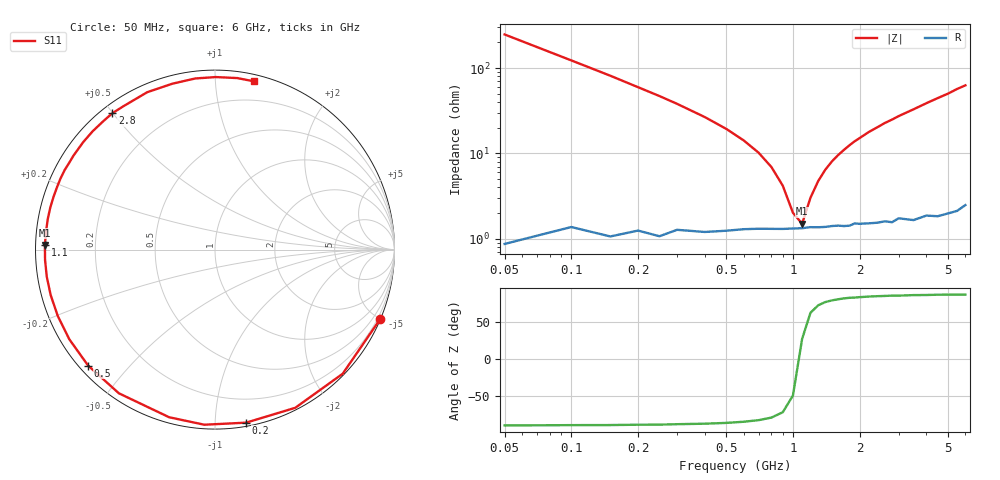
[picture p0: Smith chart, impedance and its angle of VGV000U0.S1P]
! Infineon Technologies  Discrete & RF Semiconductors
! BB 831
! Si Tuning Diode in SOD323
! VR = 0 V
! S-Parameters:  July  1999
# GHz  S  MA  R  50
!  f  S11
! GHz  MAG  ANG
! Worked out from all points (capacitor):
!   34 points, 50 MHz to 6 GHz, reference 50 ohm
!   read as one part to ground: C = 12.8 pF near 50 MHz
!   lowest |Z| = 1.5 ohm at 1.1 GHz (marker M1)
!   series resonance near 1.069 GHz, so ESL is about 1.7 nH
!   S11 on the Smith chart (normalised r, x): 50 MHz: 0.02, -4.96; 200 MHz: 0.02, -1.20; 500 MHz: 0.02, -0.39; 1.1 GHz: 0.03, +0.01; 2.8 GHz: 0.03, +0.50; 6 GHz: 0.05, +1.26
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0.05  0.9986 -22.8
0.1  0.9922 -44.2
0.15  0.9884 -63.1
0.2  0.9797 -79.8
0.25  0.9775 -93.5
0.3  0.9683 -105.3
0.4  0.9633 -123.8
0.5  0.9577 -137.6
0.6  0.9531 -148.4
0.7  0.9508 -157.1
0.8  0.9499 -164.5
0.9  0.9494 -170.9
1.1  0.9481 178.4
1.2  0.9468 173.8
1.4  0.9472 165.6
1.6  0.9464 158.5
1.9  0.9453 149.1
2.2  0.9475 140.8
2.4  0.9483 136.0
2.6  0.9483 131.1
2.8  0.9511 127.0
3  0.9479 122.6
3.5  0.9548 113.3
4  0.9543 104.4
4.5  0.9598 96.6
5  0.9613 89.8
5.5  0.9637 82.6
6  0.9622 77.0
